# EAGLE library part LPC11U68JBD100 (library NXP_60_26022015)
32-bit ARM Cortex-M0+ microcontroller; up to 256 kB flash and 36 kB SRAM; 4 kB EEPROM; USB; 12-bit ADC The LPC11U6x are an ARM Cortex-M0+ based, low-cost 32-bit MCU family operating at CPU frequencies of up to 50 MHz. The LPC11U6x support up to 256 kB of flash memory, a 4 kB EEPROM, and 36 kB of SRAM. The ARM Cortex-M0+ is an easy-to-use, energy-efficient core using a two-stage pipeline and fast single-cycle I/O access. The peripheral complement of the LPC11U6x includes a DMA controller, a CRC engine, one full-speed USB device controller with XTAL-less low-speed mode, two I2C-bus interfaces, up to five USARTs, two SSP interfaces, PWM/timer subsystem with six configurable multi-purpose timers, a Real-Time Clock, one 12-bit ADC, temperature sensor, function-configurable I/O ports, and up to 80 general-purpose I/O pins. AAL Eindhoven MK
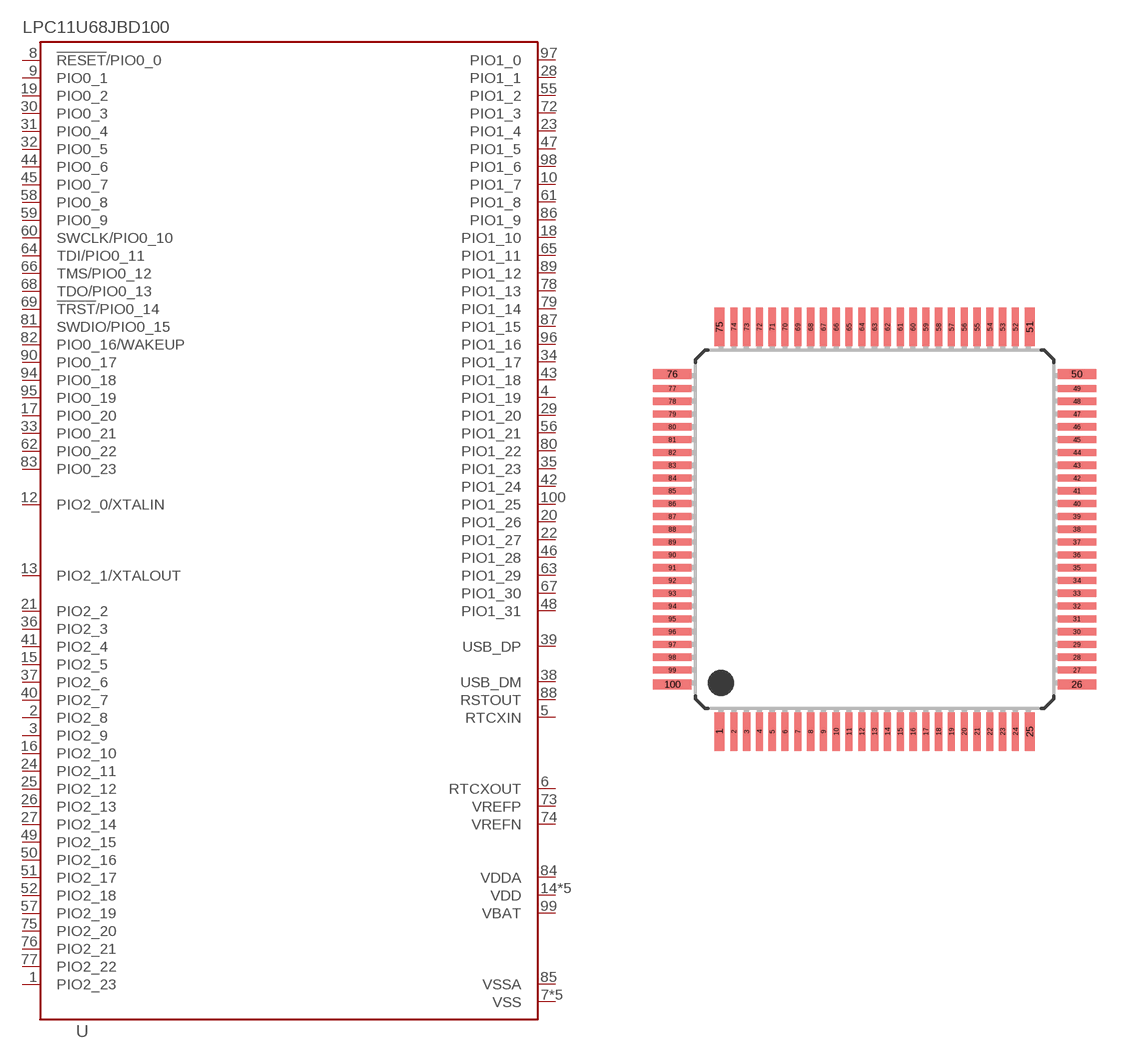
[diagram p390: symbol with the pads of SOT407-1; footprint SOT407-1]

Designator prefix U

## LPC11U68JBD100  [SOT407-1]
1  PIO2_23
2  PIO2_8
3  PIO2_9
4  PIO1_19
5  RTCXIN
6  RTCXOUT
7  VSS
8  !RESET!/PIO0_0
9  PIO0_1
10  PIO1_7
11  VSS
12  PIO2_0/XTALIN
13  PIO2_1/XTALOUT
14  VDD
15  PIO2_5
16  PIO2_10
17  PIO0_20
18  PIO1_10
19  PIO0_2
20  PIO1_26
21  PIO2_2
22  PIO1_27
23  PIO1_4
24  PIO2_11
25  PIO2_12
26  PIO2_13
27  PIO2_14
28  PIO1_1
29  PIO1_20
30  PIO0_3
31  PIO0_4
32  PIO0_5
33  PIO0_21
34  PIO1_17
35  PIO1_23
36  PIO2_3
37  PIO2_6
38  USB_DM
39  USB_DP
40  PIO2_7
41  PIO2_4
42  PIO1_24
43  PIO1_18
44  PIO0_6
45  PIO0_7
46  PIO1_28
47  PIO1_5
48  PIO1_31
49  PIO2_15
50  PIO2_16
51  PIO2_17
52  PIO2_18
53  VSS
54  VDD
55  PIO1_2
56  PIO1_21
57  PIO2_19
58  PIO0_8
59  PIO0_9
60  SWCLK/PIO0_10
61  PIO1_8
62  PIO0_22
63  PIO1_29
64  TDI/PIO0_11
65  PIO1_11
66  TMS/PIO0_12
67  PIO1_30
68  TDO/PIO0_13
69  !TRST!/PIO0_14
70  VSS
71  VDD
72  PIO1_3
73  VREFP
74  VREFN
75  PIO2_20
76  PIO2_21
77  PIO2_22
78  PIO1_13
79  PIO1_14
80  PIO1_22
81  SWDIO/PIO0_15
82  PIO0_16/WAKEUP
83  PIO0_23
84  VDDA
85  VSSA
86  PIO1_9
87  PIO1_15
88  RSTOUT
89  PIO1_12
90  PIO0_17
91  VSS
92  VDD
93  VDD
94  PIO0_18
95  PIO0_19
96  PIO1_16
97  PIO1_0
98  PIO1_6
99  VBAT
100  PIO1_25

## Footprint SOT407-1 (pad centres in mm)
SOT407-1 LQFP100: plastic low profile quad flat package; 100 leads; body 14 x 14 x 1.4 mm JEDEC: MS-026 IEC: 136E20
smd 0.4 x 1.5: 1 -6.06,-7.9; 25 6.06,-7.9; 51 6.06,7.9; 75 -6.06,7.9
smd 0.28 x 1.5: 2 -5.5,-7.9; 3 -5,-7.9; 4 -4.5,-7.9; 5 -4,-7.9; 6 -3.5,-7.9; 7 -3,-7.9; 8 -2.5,-7.9; 9 -2,-7.9; 10 -1.5,-7.9; 11 -1,-7.9; 12 -0.5,-7.9; 13 0,-7.9; 14 0.5,-7.9; 15 1,-7.9; 16 1.5,-7.9; 17 2,-7.9; 18 2.5,-7.9; 19 3,-7.9; 20 3.5,-7.9; 21 4,-7.9; 22 4.5,-7.9; 23 5,-7.9; 24 5.5,-7.9; 52 5.5,7.9; 53 5,7.9; 54 4.5,7.9; 55 4,7.9; 56 3.5,7.9; 57 3,7.9; 58 2.5,7.9; 59 2,7.9; 60 1.5,7.9; 61 1,7.9; 62 0.5,7.9; 63 0,7.9; 64 -0.5,7.9; 65 -1,7.9; 66 -1.5,7.9; 67 -2,7.9; 68 -2.5,7.9; 69 -3,7.9; 70 -3.5,7.9; 71 -4,7.9; 72 -4.5,7.9; 73 -5,7.9; 74 -5.5,7.9
smd 1.5 x 0.4: 26 7.9,-6.06; 50 7.9,6.06; 76 -7.9,6.06; 100 -7.9,-6.06
smd 1.5 x 0.28: 27 7.9,-5.5; 28 7.9,-5; 29 7.9,-4.5; 30 7.9,-4; 31 7.9,-3.5; 32 7.9,-3; 33 7.9,-2.5; 34 7.9,-2; 35 7.9,-1.5; 36 7.9,-1; 37 7.9,-0.5; 38 7.9,0; 39 7.9,0.5; 40 7.9,1; 41 7.9,1.5; 42 7.9,2; 43 7.9,2.5; 44 7.9,3; 45 7.9,3.5; 46 7.9,4; 47 7.9,4.5; 48 7.9,5; 49 7.9,5.5; 77 -7.9,5.5; 78 -7.9,5; 79 -7.9,4.5; 80 -7.9,4; 81 -7.9,3.5; 82 -7.9,3; 83 -7.9,2.5; 84 -7.9,2; 85 -7.9,1.5; 86 -7.9,1; 87 -7.9,0.5; 88 -7.9,0; 89 -7.9,-0.5; 90 -7.9,-1; 91 -7.9,-1.5; 92 -7.9,-2; 93 -7.9,-2.5; 94 -7.9,-3; 95 -7.9,-3.5; 96 -7.9,-4; 97 -7.9,-4.5; 98 -7.9,-5; 99 -7.9,-5.5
